(* Logix 5000 AddOnInstructionDefinition export YAI_Assy_70_71_20_21_EIP_Hz; software revision 17.00 *)

ADD_ON_INSTRUCTION YAI_Assy_70_71_20_21_EIP_Hz   (* revision 1.0, vendor Yaskawa America, Inc. *)
// YAI Assembly 70/71 and 20/21
// Help:
// This add-on instruction is for use with input assemblie 70 or 71 and output assemblies 20 or 21.
// Node_Input_Assy is defined as the node's input assembly integer array.
// Node_Output_Assy is defined as the node's output assembly integer array.
VAR_IN_OUT
   Node_Input_Assy : AB:ETHERNET_MODULE_INT_4Bytes:I:0; {required}   // Input assembly words
   Node_Output_Assy : AB:ETHERNET_MODULE_INT_4Bytes:O:0; {required}   // Output assembly words
END_VAR
VAR_INPUT
   RunFwd : BOOL; {visible}   // Forward run command
   RunRev : BOOL; {visible}   // Reverse run command
   FaultReset : BOOL; {visible}   // Fault reset command
   Net_Control : BOOL;   // Network control bit to switch between b1-02 setting and network.
   Net_Ref : BOOL;   // Network reference bit to switch between b1-01 setting and network.
   Freq_Ref : REAL; {visible}   // Frequency reference command in Hz (xx.xx resolution)
END_VAR
VAR_OUTPUT
   Faulted : BOOL; {visible}   // Drive faulted status bit
   Warning : BOOL; {visible}   // Drive warning (alarm) status bit
   RunningFwd : BOOL; {visible}   // Drive running forward status bit
   RunningRev : BOOL; {visible}   // Drive running reverse status bit
   Ready : BOOL; {visible}   // Drive ready status bit
   NetRefStatus : BOOL; {visible}   // Drive network reference status bit (1 = reference coming from network)
   NetCtrlStatus : BOOL; {visible}   // Drive network run source status bit (1 = source coming from network)
   At_Speed : BOOL; {visible}   // Drive at commanded speed status bit
   Output_Freq : REAL; {visible}   // Drive output frequency in Hz (xx.xx resolution)
END_VAR
VAR
   FRef_Convert : DINT;
   FOut_Convert : REAL;
   FOut_Temp : REAL;
   Fault_Reset_Timer : TIMER := (PRE := 250);
END_VAR

ROUTINE Logic   (* ladder *)
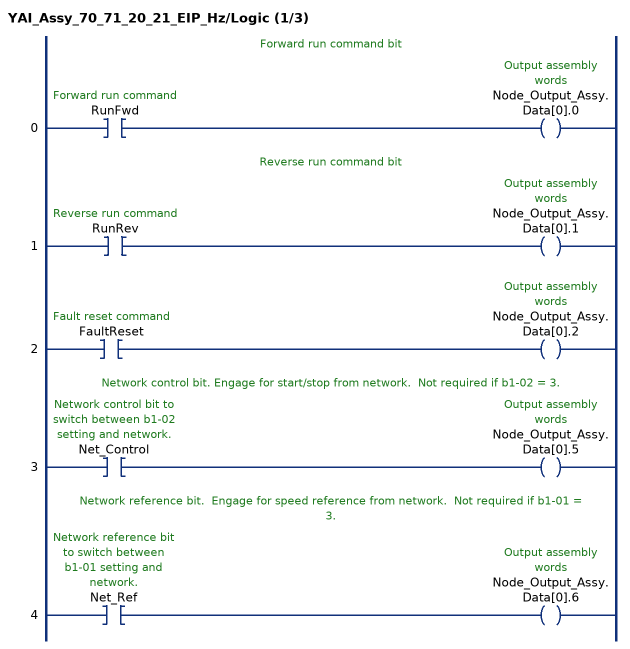
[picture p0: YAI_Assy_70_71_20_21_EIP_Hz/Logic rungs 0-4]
   // Forward run command bit
   0: XIC(RunFwd)OTE(Node_Output_Assy.Data[0].0);
   // Reverse run command bit
   1: XIC(RunRev)OTE(Node_Output_Assy.Data[0].1);
   2: XIC(FaultReset)OTE(Node_Output_Assy.Data[0].2);
   // Network control bit. Engage for start/stop from network.  Not required if b1-02 = 3.
   3: XIC(Net_Control)OTE(Node_Output_Assy.Data[0].5);
   // Network reference bit.  Engage for speed reference from network.  Not required if b1-01 = 3.
   4: XIC(Net_Ref)OTE(Node_Output_Assy.Data[0].6);
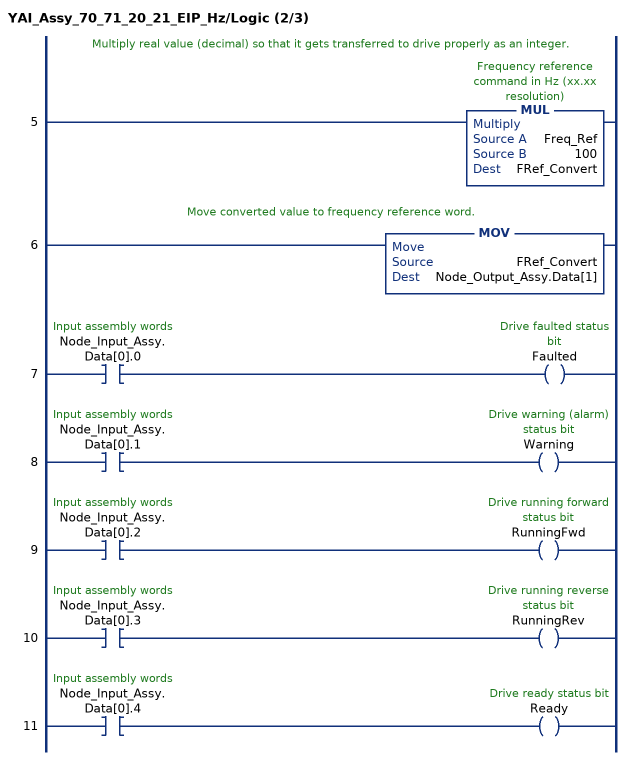
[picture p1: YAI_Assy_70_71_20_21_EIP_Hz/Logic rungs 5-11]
   // Multiply real value (decimal) so that it gets transferred to drive properly as an integer.
   5: MUL(Freq_Ref,100,FRef_Convert);
   // Move converted value to frequency reference word.
   6: MOV(FRef_Convert,Node_Output_Assy.Data[1]);
   7: XIC(Node_Input_Assy.Data[0].0)OTE(Faulted);
   8: XIC(Node_Input_Assy.Data[0].1)OTE(Warning);
   9: XIC(Node_Input_Assy.Data[0].2)OTE(RunningFwd);
   10: XIC(Node_Input_Assy.Data[0].3)OTE(RunningRev);
   11: XIC(Node_Input_Assy.Data[0].4)OTE(Ready);
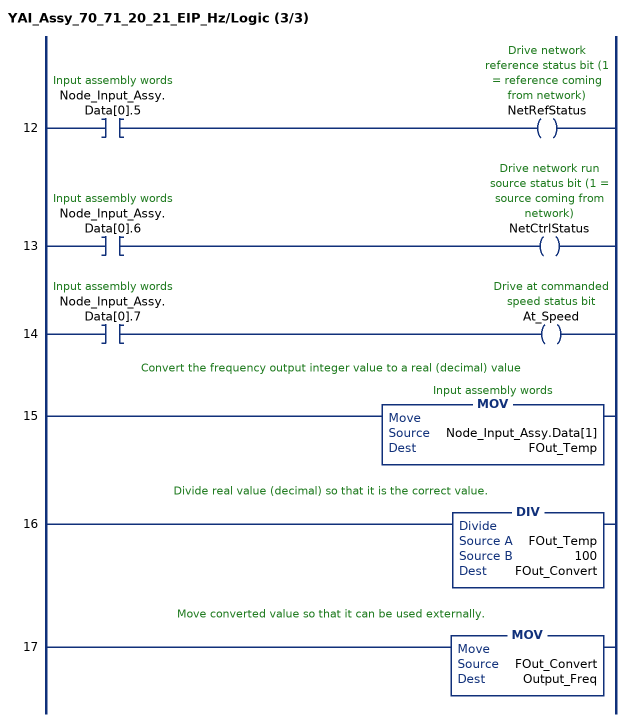
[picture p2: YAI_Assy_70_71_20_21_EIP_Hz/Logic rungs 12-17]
   12: XIC(Node_Input_Assy.Data[0].5)OTE(NetRefStatus);
   13: XIC(Node_Input_Assy.Data[0].6)OTE(NetCtrlStatus);
   14: XIC(Node_Input_Assy.Data[0].7)OTE(At_Speed);
   // Convert the frequency output integer value to a real (decimal) value
   15: MOV(Node_Input_Assy.Data[1],FOut_Temp);
   // Divide real value (decimal) so that it is the correct value.
   16: DIV(FOut_Temp,100,FOut_Convert);
   // Move converted value so that it can be used externally.
   17: MOV(FOut_Convert,Output_Freq);
END_ROUTINE
END_ADD_ON_INSTRUCTION
